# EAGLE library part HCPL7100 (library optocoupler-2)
HEWLETT PACKARD OPTO COUPLER
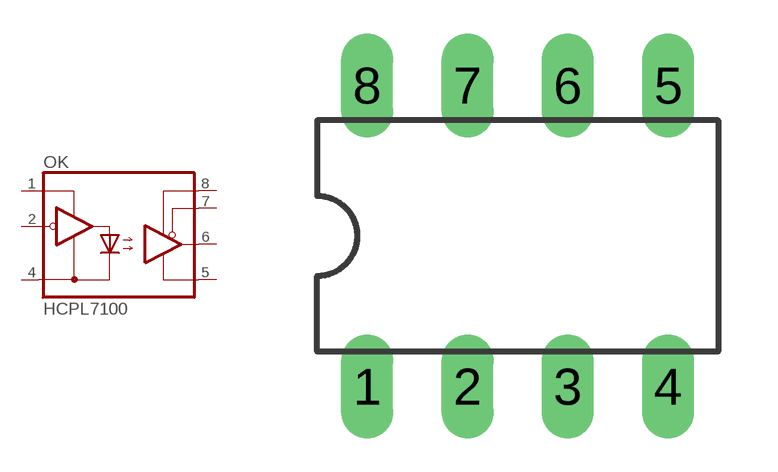
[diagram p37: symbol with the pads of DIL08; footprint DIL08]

Designator prefix OK

## HCPL7100  [DIL08]
1  VDD1  pas
2  VI  pas
4  GND1  pas
5  GND2  pas
6  VO  pas
7  VE  pas
8  VDD2  pas

## Footprint DIL08 (pad centres in mm)
Dual In Line Package
drill 0.813 long: 1 -3.81,-3.81; 2 -1.27,-3.81; 3 1.27,-3.81; 4 3.81,-3.81; 5 3.81,3.81; 6 1.27,3.81; 7 -1.27,3.81; 8 -3.81,3.81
